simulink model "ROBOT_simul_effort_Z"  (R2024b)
settings: Solver=VariableStepAuto  StartTime=0.0  StopTime=5  RelTol=1e-3
undefined symbols (not defined in the file): a, ARRIERE_Defaut_sldprt, avant01_Defaut_sldprt, avant02_Defaut_sldprt, avant03_Defaut_sldprt, avant1_Defaut_sldprt, AXE, BASE_Defaut_sldprt, BIELLE, BIELLE_Defaut_sldprt, BRAS_Defaut_sldprt, bras_Defaut_sldprt, C_Realiste_sldprt, CABLE_Defaut_sldprt, cable_Defaut_sldprt, CACHE_Defaut_sldprt, CARTE, carte_Defaut_sldprt, CARTER, carter, CHC, CODEUR_Defaut_sldprt, cruciforme, cylindrique, deg, Drive, Fichiers, Fichiers_Matlab_sujetA, FIXATION, fixation_Defaut_sldprt, H, HEXAGONALE_Defaut_sldprt, joint_Defaut_sldprt, kg, m, M4, M4_Defaut_sldprt, manette1_Defaut_sldprt, manette2_Defaut_sldprt, MATLAB, Matlab, matlab_Defaut_sldprt, mm, modif, MOTEUR_Defaut_sldprt, N, NEZ_Defaut_sldprt, nom, palier, PARALLELOGRAMME_Defaut_sldprt, petite, plaque, rad, Ressort, Rondelle, ROTOR_Defaut_sldprt, s, SET, simple, socle_Defaut_sldprt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
libraries: sm_lib x463, fl_lib x45, nesl_utility x27, simulink x2
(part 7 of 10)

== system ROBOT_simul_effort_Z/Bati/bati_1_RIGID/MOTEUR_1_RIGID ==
  ReferenceFrame : sm_lib/Frames and Transforms/Reference Frame
  Solid : sm_lib/Body Elements/File Solid  ExtGeomFileName=/MATLAB Drive/Fichiers_Matlab_sujetA/Fichiers Matlab/STL/MOTEUR_Defaut_sldprt.STL  UnitType=Custom  ExtGeomFileUnits=mm  StepReaderType=HEX  ExportConvexHullGeometry=off  InertiaType=Custom  BasedOnType=Density  Density=1000  DensityUnits=kg/(m^3)  Mass=0.064287172119754279  MassUnits=kg  CenterOfMass=[0 32.927342518193171 0]  CenterOfMassUnits=mm  MomentsOfInertia=[23.361167142247837 11.499741081133124 23.353822804254591]  MomentsOfInertiaUnits=kg*mm^2  ProductsOfInertia=[0 0 0]  ProductsOfInertiaUnits=kg*mm^2  GraphicType=FromGeometry  MarkerShape=Sphere  MarkerSize=10  GraphicVisPropType=SimpleVisualProperties  GraphicDiffuseColor=[0.792156862745098 0.81960784313725488 0.93333333333333335]  GraphicOpacity=1  GraphicSpecularColor=[0.5 0.5 0.5 1.0]  GraphicAmbientColor=[0.15 0.15 0.15 1.0]  GraphicEmissiveColor=[0.0 0.0 0.0 1.0]  GraphicShininess=75  DoExposeReferenceFrame=on  SerializedFrames=<Frames/>
  F : PMIOPort  Side=Left
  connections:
  Solid/RConn1 -- ReferenceFrame/RConn1 -- F/RConn1

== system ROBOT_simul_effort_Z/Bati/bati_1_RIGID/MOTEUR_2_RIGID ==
  ReferenceFrame : sm_lib/Frames and Transforms/Reference Frame
  Solid : sm_lib/Body Elements/File Solid  ExtGeomFileName=/MATLAB Drive/Fichiers_Matlab_sujetA/Fichiers Matlab/STL/MOTEUR_Defaut_sldprt.STL  UnitType=Custom  ExtGeomFileUnits=mm  StepReaderType=HEX  ExportConvexHullGeometry=off  InertiaType=Custom  BasedOnType=Density  Density=1000  DensityUnits=kg/(m^3)  Mass=0.064287172119754279  MassUnits=kg  CenterOfMass=[0 32.927342518193171 0]  CenterOfMassUnits=mm  MomentsOfInertia=[23.361167142247837 11.499741081133124 23.353822804254591]  MomentsOfInertiaUnits=kg*mm^2  ProductsOfInertia=[0 0 0]  ProductsOfInertiaUnits=kg*mm^2  GraphicType=FromGeometry  MarkerShape=Sphere  MarkerSize=10  GraphicVisPropType=SimpleVisualProperties  GraphicDiffuseColor=[0.792156862745098 0.81960784313725488 0.93333333333333335]  GraphicOpacity=1  GraphicSpecularColor=[0.5 0.5 0.5 1.0]  GraphicAmbientColor=[0.15 0.15 0.15 1.0]  GraphicEmissiveColor=[0.0 0.0 0.0 1.0]  GraphicShininess=75  DoExposeReferenceFrame=on  SerializedFrames=<Frames/>
  F : PMIOPort  Side=Left
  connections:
  Solid/RConn1 -- ReferenceFrame/RConn1 -- F/RConn1

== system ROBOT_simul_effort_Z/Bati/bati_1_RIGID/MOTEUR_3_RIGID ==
  ReferenceFrame : sm_lib/Frames and Transforms/Reference Frame
  Solid : sm_lib/Body Elements/File Solid  ExtGeomFileName=/MATLAB Drive/Fichiers_Matlab_sujetA/Fichiers Matlab/STL/MOTEUR_Defaut_sldprt.STL  UnitType=Custom  ExtGeomFileUnits=mm  StepReaderType=HEX  ExportConvexHullGeometry=off  InertiaType=Custom  BasedOnType=Density  Density=1000  DensityUnits=kg/(m^3)  Mass=0.064287172119754279  MassUnits=kg  CenterOfMass=[0 32.927342518193171 0]  CenterOfMassUnits=mm  MomentsOfInertia=[23.361167142247837 11.499741081133124 23.353822804254591]  MomentsOfInertiaUnits=kg*mm^2  ProductsOfInertia=[0 0 0]  ProductsOfInertiaUnits=kg*mm^2  GraphicType=FromGeometry  MarkerShape=Sphere  MarkerSize=10  GraphicVisPropType=SimpleVisualProperties  GraphicDiffuseColor=[0.792156862745098 0.81960784313725488 0.93333333333333335]  GraphicOpacity=1  GraphicSpecularColor=[0.5 0.5 0.5 1.0]  GraphicAmbientColor=[0.15 0.15 0.15 1.0]  GraphicEmissiveColor=[0.0 0.0 0.0 1.0]  GraphicShininess=75  DoExposeReferenceFrame=on  SerializedFrames=<Frames/>
  F : PMIOPort  Side=Left
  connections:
  Solid/RConn1 -- ReferenceFrame/RConn1 -- F/RConn1

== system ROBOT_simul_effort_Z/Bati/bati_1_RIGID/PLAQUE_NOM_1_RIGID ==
  ReferenceFrame : sm_lib/Frames and Transforms/Reference Frame
  Solid : sm_lib/Body Elements/File Solid  ExtGeomFileName=/MATLAB Drive/Fichiers_Matlab_sujetA/Fichiers Matlab/STL/plaque nom simple-1.STL  UnitType=Custom  ExtGeomFileUnits=mm  StepReaderType=HEX  ExportConvexHullGeometry=off  InertiaType=Custom  BasedOnType=Density  Density=1000  DensityUnits=kg/(m^3)  Mass=0.00027200040900533893  MassUnits=kg  CenterOfMass=[-0.0026353545106053435 115.22134035146432 0.049293923597036424]  CenterOfMassUnits=mm  MomentsOfInertia=[0.063569474995042688 0.063782951879047547 0.12735197367307241]  MomentsOfInertiaUnits=kg*mm^2  ProductsOfInertia=[2.9045793709905346e-07 6.1711886469806189e-08 2.2164861893284939e-05]  ProductsOfInertiaUnits=kg*mm^2  GraphicType=FromGeometry  MarkerShape=Sphere  MarkerSize=10  GraphicVisPropType=SimpleVisualProperties  GraphicDiffuseColor=[1.0 1.0 1.0]  GraphicOpacity=1  GraphicSpecularColor=[0.5 0.5 0.5 1.0]  GraphicAmbientColor=[0.15 0.15 0.15 1.0]  GraphicEmissiveColor=[0.0 0.0 0.0 1.0]  GraphicShininess=75  DoExposeReferenceFrame=on  SerializedFrames=<Frames/>
  F : PMIOPort  Side=Left
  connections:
  Solid/RConn1 -- ReferenceFrame/RConn1 -- F/RConn1

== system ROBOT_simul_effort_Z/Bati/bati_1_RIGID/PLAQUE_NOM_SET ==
  ReferenceFrame : sm_lib/Frames and Transforms/Reference Frame
  Solid : sm_lib/Body Elements/File Solid  ExtGeomFileName=/MATLAB Drive/Fichiers_Matlab_sujetA/Fichiers Matlab/STL/plaque nom SET-1.STL  UnitType=Custom  ExtGeomFileUnits=mm  StepReaderType=HEX  ExportConvexHullGeometry=off  InertiaType=Custom  BasedOnType=Density  Density=1000  DensityUnits=kg/(m^3)  Mass=0.00027200040900533893  MassUnits=kg  CenterOfMass=[-0.0026353545106053435 115.22134035146432 0.049293923597036424]  CenterOfMassUnits=mm  MomentsOfInertia=[0.063569474995042688 0.063782951879047547 0.12735197367307241]  MomentsOfInertiaUnits=kg*mm^2  ProductsOfInertia=[2.9045793709905346e-07 6.1711886469806189e-08 2.2164861893284939e-05]  ProductsOfInertiaUnits=kg*mm^2  GraphicType=FromGeometry  MarkerShape=Sphere  MarkerSize=10  GraphicVisPropType=SimpleVisualProperties  GraphicDiffuseColor=[0.2 0.2 1.0]  GraphicOpacity=1  GraphicSpecularColor=[0.5 0.5 0.5 1.0]  GraphicAmbientColor=[0.15 0.15 0.15 1.0]  GraphicEmissiveColor=[0.0 0.0 0.0 1.0]  GraphicShininess=75  DoExposeReferenceFrame=on  SerializedFrames=<Frames/>
  F : PMIOPort  Side=Left
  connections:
  F/RConn1 -- ReferenceFrame/RConn1 -- Solid/RConn1

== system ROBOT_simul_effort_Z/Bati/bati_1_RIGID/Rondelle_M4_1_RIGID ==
  ReferenceFrame : sm_lib/Frames and Transforms/Reference Frame
  Solid : sm_lib/Body Elements/File Solid  ExtGeomFileName=/MATLAB Drive/Fichiers_Matlab_sujetA/Fichiers Matlab/STL/Rondelle M4_Defaut_sldprt.STL  UnitType=Custom  ExtGeomFileUnits=mm  StepReaderType=HEX  ExportConvexHullGeometry=off  InertiaType=Custom  BasedOnType=Density  Density=1000  DensityUnits=kg/(m^3)  Mass=4.0840704496667297e-05  MassUnits=kg  CenterOfMass=[0 0.39999999999999991 0]  CenterOfMassUnits=mm  MomentsOfInertia=[0.00024977494191753434 0.00049519354202209084 0.00024977494191753439]  MomentsOfInertiaUnits=kg*mm^2  ProductsOfInertia=[0 0 0]  ProductsOfInertiaUnits=kg*mm^2  GraphicType=FromGeometry  MarkerShape=Sphere  MarkerSize=10  GraphicVisPropType=SimpleVisualProperties  GraphicDiffuseColor=[0.792156862745098 0.81960784313725488 0.93333333333333335]  GraphicOpacity=1  GraphicSpecularColor=[0.5 0.5 0.5 1.0]  GraphicAmbientColor=[0.15 0.15 0.15 1.0]  GraphicEmissiveColor=[0.0 0.0 0.0 1.0]  GraphicShininess=75  DoExposeReferenceFrame=on  SerializedFrames=<Frames/>
  F : PMIOPort  Side=Left
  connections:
  Solid/RConn1 -- ReferenceFrame/RConn1 -- F/RConn1

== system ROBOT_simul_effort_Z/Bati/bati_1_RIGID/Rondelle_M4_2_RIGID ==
  ReferenceFrame : sm_lib/Frames and Transforms/Reference Frame
  Solid : sm_lib/Body Elements/File Solid  ExtGeomFileName=/MATLAB Drive/Fichiers_Matlab_sujetA/Fichiers Matlab/STL/Rondelle M4_Defaut_sldprt.STL  UnitType=Custom  ExtGeomFileUnits=mm  StepReaderType=HEX  ExportConvexHullGeometry=off  InertiaType=Custom  BasedOnType=Density  Density=1000  DensityUnits=kg/(m^3)  Mass=4.0840704496667297e-05  MassUnits=kg  CenterOfMass=[0 0.39999999999999991 0]  CenterOfMassUnits=mm  MomentsOfInertia=[0.00024977494191753434 0.00049519354202209084 0.00024977494191753439]  MomentsOfInertiaUnits=kg*mm^2  ProductsOfInertia=[0 0 0]  ProductsOfInertiaUnits=kg*mm^2  GraphicType=FromGeometry  MarkerShape=Sphere  MarkerSize=10  GraphicVisPropType=SimpleVisualProperties  GraphicDiffuseColor=[0.792156862745098 0.81960784313725488 0.93333333333333335]  GraphicOpacity=1  GraphicSpecularColor=[0.5 0.5 0.5 1.0]  GraphicAmbientColor=[0.15 0.15 0.15 1.0]  GraphicEmissiveColor=[0.0 0.0 0.0 1.0]  GraphicShininess=75  DoExposeReferenceFrame=on  SerializedFrames=<Frames/>
  F : PMIOPort  Side=Left
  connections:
  Solid/RConn1 -- ReferenceFrame/RConn1 -- F/RConn1

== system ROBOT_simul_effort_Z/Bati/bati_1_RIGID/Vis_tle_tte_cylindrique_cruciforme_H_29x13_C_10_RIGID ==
  ReferenceFrame : sm_lib/Frames and Transforms/Reference Frame
  Solid : sm_lib/Body Elements/File Solid  ExtGeomFileName=/MATLAB Drive/Fichiers_Matlab_sujetA/Fichiers Matlab/STL/Vis a tole tete cylindrique cruciforme H 2-9x13 - C_Realiste_sldprt.STL  UnitType=Custom  ExtGeomFileUnits=mm  StepReaderType=HEX  ExportConvexHullGeometry=off  InertiaType=Custom  BasedOnType=Density  Density=1000  DensityUnits=kg/(m^3)  Mass=8.3821869835456372e-05  MassUnits=kg  CenterOfMass=[4.9478681581074904 0.00064910481891303923 -0.0013634218224953438]  CenterOfMassUnits=mm  MomentsOfInertia=[0.00016543197172893975 0.0014334630955093895 0.0014333390308476422]  MomentsOfInertiaUnits=kg*mm^2  ProductsOfInertia=[-5.4062904633677868e-09 -1.3111174919527308e-07 6.0713893531177014e-07]  ProductsOfInertiaUnits=kg*mm^2  GraphicType=FromGeometry  MarkerShape=Sphere  MarkerSize=10  GraphicVisPropType=SimpleVisualProperties  GraphicDiffuseColor=[0.75294117647058822 0.75294117647058822 0.75294117647058822]  GraphicOpacity=1  GraphicSpecularColor=[0.5 0.5 0.5 1.0]  GraphicAmbientColor=[0.15 0.15 0.15 1.0]  GraphicEmissiveColor=[0.0 0.0 0.0 1.0]  GraphicShininess=75  DoExposeReferenceFrame=on  SerializedFrames=<Frames/>
  F : PMIOPort  Side=Left
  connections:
  Solid/RConn1 -- ReferenceFrame/RConn1 -- F/RConn1

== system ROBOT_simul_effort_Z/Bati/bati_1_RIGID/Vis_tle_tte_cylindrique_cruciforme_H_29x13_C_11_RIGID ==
  ReferenceFrame : sm_lib/Frames and Transforms/Reference Frame
  Solid : sm_lib/Body Elements/File Solid  ExtGeomFileName=/MATLAB Drive/Fichiers_Matlab_sujetA/Fichiers Matlab/STL/Vis a tole tete cylindrique cruciforme H 2-9x13 - C_Realiste_sldprt.STL  UnitType=Custom  ExtGeomFileUnits=mm  StepReaderType=HEX  ExportConvexHullGeometry=off  InertiaType=Custom  BasedOnType=Density  Density=1000  DensityUnits=kg/(m^3)  Mass=8.3821869835456372e-05  MassUnits=kg  CenterOfMass=[4.9478681581074904 0.00064910481891303923 -0.0013634218224953438]  CenterOfMassUnits=mm  MomentsOfInertia=[0.00016543197172893975 0.0014334630955093895 0.0014333390308476422]  MomentsOfInertiaUnits=kg*mm^2  ProductsOfInertia=[-5.4062904633677868e-09 -1.3111174919527308e-07 6.0713893531177014e-07]  ProductsOfInertiaUnits=kg*mm^2  GraphicType=FromGeometry  MarkerShape=Sphere  MarkerSize=10  GraphicVisPropType=SimpleVisualProperties  GraphicDiffuseColor=[0.75294117647058822 0.75294117647058822 0.75294117647058822]  GraphicOpacity=1  GraphicSpecularColor=[0.5 0.5 0.5 1.0]  GraphicAmbientColor=[0.15 0.15 0.15 1.0]  GraphicEmissiveColor=[0.0 0.0 0.0 1.0]  GraphicShininess=75  DoExposeReferenceFrame=on  SerializedFrames=<Frames/>
  F : PMIOPort  Side=Left
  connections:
  Solid/RConn1 -- ReferenceFrame/RConn1 -- F/RConn1

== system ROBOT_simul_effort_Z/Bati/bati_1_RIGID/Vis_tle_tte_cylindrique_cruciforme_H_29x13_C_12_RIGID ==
  ReferenceFrame : sm_lib/Frames and Transforms/Reference Frame
  Solid : sm_lib/Body Elements/File Solid  ExtGeomFileName=/MATLAB Drive/Fichiers_Matlab_sujetA/Fichiers Matlab/STL/Vis a tole tete cylindrique cruciforme H 2-9x13 - C_Realiste_sldprt.STL  UnitType=Custom  ExtGeomFileUnits=mm  StepReaderType=HEX  ExportConvexHullGeometry=off  InertiaType=Custom  BasedOnType=Density  Density=1000  DensityUnits=kg/(m^3)  Mass=8.3821869835456372e-05  MassUnits=kg  CenterOfMass=[4.9478681581074904 0.00064910481891303923 -0.0013634218224953438]  CenterOfMassUnits=mm  MomentsOfInertia=[0.00016543197172893975 0.0014334630955093895 0.0014333390308476422]  MomentsOfInertiaUnits=kg*mm^2  ProductsOfInertia=[-5.4062904633677868e-09 -1.3111174919527308e-07 6.0713893531177014e-07]  ProductsOfInertiaUnits=kg*mm^2  GraphicType=FromGeometry  MarkerShape=Sphere  MarkerSize=10  GraphicVisPropType=SimpleVisualProperties  GraphicDiffuseColor=[0.75294117647058822 0.75294117647058822 0.75294117647058822]  GraphicOpacity=1  GraphicSpecularColor=[0.5 0.5 0.5 1.0]  GraphicAmbientColor=[0.15 0.15 0.15 1.0]  GraphicEmissiveColor=[0.0 0.0 0.0 1.0]  GraphicShininess=75  DoExposeReferenceFrame=on  SerializedFrames=<Frames/>
  F : PMIOPort  Side=Left
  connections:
  Solid/RConn1 -- ReferenceFrame/RConn1 -- F/RConn1

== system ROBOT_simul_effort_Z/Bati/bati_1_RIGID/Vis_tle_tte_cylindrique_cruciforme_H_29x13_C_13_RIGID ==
  ReferenceFrame : sm_lib/Frames and Transforms/Reference Frame
  Solid : sm_lib/Body Elements/File Solid  ExtGeomFileName=/MATLAB Drive/Fichiers_Matlab_sujetA/Fichiers Matlab/STL/Vis a tole tete cylindrique cruciforme H 2-9x13 - C_Realiste_sldprt.STL  UnitType=Custom  ExtGeomFileUnits=mm  StepReaderType=HEX  ExportConvexHullGeometry=off  InertiaType=Custom  BasedOnType=Density  Density=1000  DensityUnits=kg/(m^3)  Mass=8.3821869835456372e-05  MassUnits=kg  CenterOfMass=[4.9478681581074904 0.00064910481891303923 -0.0013634218224953438]  CenterOfMassUnits=mm  MomentsOfInertia=[0.00016543197172893975 0.0014334630955093895 0.0014333390308476422]  MomentsOfInertiaUnits=kg*mm^2  ProductsOfInertia=[-5.4062904633677868e-09 -1.3111174919527308e-07 6.0713893531177014e-07]  ProductsOfInertiaUnits=kg*mm^2  GraphicType=FromGeometry  MarkerShape=Sphere  MarkerSize=10  GraphicVisPropType=SimpleVisualProperties  GraphicDiffuseColor=[0.75294117647058822 0.75294117647058822 0.75294117647058822]  GraphicOpacity=1  GraphicSpecularColor=[0.5 0.5 0.5 1.0]  GraphicAmbientColor=[0.15 0.15 0.15 1.0]  GraphicEmissiveColor=[0.0 0.0 0.0 1.0]  GraphicShininess=75  DoExposeReferenceFrame=on  SerializedFrames=<Frames/>
  F : PMIOPort  Side=Left
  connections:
  Solid/RConn1 -- ReferenceFrame/RConn1 -- F/RConn1

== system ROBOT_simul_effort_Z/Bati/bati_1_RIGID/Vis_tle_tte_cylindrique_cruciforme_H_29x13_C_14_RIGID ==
  ReferenceFrame : sm_lib/Frames and Transforms/Reference Frame
  Solid : sm_lib/Body Elements/File Solid  ExtGeomFileName=/MATLAB Drive/Fichiers_Matlab_sujetA/Fichiers Matlab/STL/Vis a tole tete cylindrique cruciforme H 2-9x13 - C_Realiste_sldprt.STL  UnitType=Custom  ExtGeomFileUnits=mm  StepReaderType=HEX  ExportConvexHullGeometry=off  InertiaType=Custom  BasedOnType=Density  Density=1000  DensityUnits=kg/(m^3)  Mass=8.3821869835456372e-05  MassUnits=kg  CenterOfMass=[4.9478681581074904 0.00064910481891303923 -0.0013634218224953438]  CenterOfMassUnits=mm  MomentsOfInertia=[0.00016543197172893975 0.0014334630955093895 0.0014333390308476422]  MomentsOfInertiaUnits=kg*mm^2  ProductsOfInertia=[-5.4062904633677868e-09 -1.3111174919527308e-07 6.0713893531177014e-07]  ProductsOfInertiaUnits=kg*mm^2  GraphicType=FromGeometry  MarkerShape=Sphere  MarkerSize=10  GraphicVisPropType=SimpleVisualProperties  GraphicDiffuseColor=[0.75294117647058822 0.75294117647058822 0.75294117647058822]  GraphicOpacity=1  GraphicSpecularColor=[0.5 0.5 0.5 1.0]  GraphicAmbientColor=[0.15 0.15 0.15 1.0]  GraphicEmissiveColor=[0.0 0.0 0.0 1.0]  GraphicShininess=75  DoExposeReferenceFrame=on  SerializedFrames=<Frames/>
  F : PMIOPort  Side=Left
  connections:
  Solid/RConn1 -- ReferenceFrame/RConn1 -- F/RConn1

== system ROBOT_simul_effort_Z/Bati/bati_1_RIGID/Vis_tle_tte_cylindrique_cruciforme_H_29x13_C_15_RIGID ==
  ReferenceFrame : sm_lib/Frames and Transforms/Reference Frame
  Solid : sm_lib/Body Elements/File Solid  ExtGeomFileName=/MATLAB Drive/Fichiers_Matlab_sujetA/Fichiers Matlab/STL/Vis a tole tete cylindrique cruciforme H 2-9x13 - C_Realiste_sldprt.STL  UnitType=Custom  ExtGeomFileUnits=mm  StepReaderType=HEX  ExportConvexHullGeometry=off  InertiaType=Custom  BasedOnType=Density  Density=1000  DensityUnits=kg/(m^3)  Mass=8.3821869835456372e-05  MassUnits=kg  CenterOfMass=[4.9478681581074904 0.00064910481891303923 -0.0013634218224953438]  CenterOfMassUnits=mm  MomentsOfInertia=[0.00016543197172893975 0.0014334630955093895 0.0014333390308476422]  MomentsOfInertiaUnits=kg*mm^2  ProductsOfInertia=[-5.4062904633677868e-09 -1.3111174919527308e-07 6.0713893531177014e-07]  ProductsOfInertiaUnits=kg*mm^2  GraphicType=FromGeometry  MarkerShape=Sphere  MarkerSize=10  GraphicVisPropType=SimpleVisualProperties  GraphicDiffuseColor=[0.75294117647058822 0.75294117647058822 0.75294117647058822]  GraphicOpacity=1  GraphicSpecularColor=[0.5 0.5 0.5 1.0]  GraphicAmbientColor=[0.15 0.15 0.15 1.0]  GraphicEmissiveColor=[0.0 0.0 0.0 1.0]  GraphicShininess=75  DoExposeReferenceFrame=on  SerializedFrames=<Frames/>
  F : PMIOPort  Side=Left
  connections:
  Solid/RConn1 -- ReferenceFrame/RConn1 -- F/RConn1

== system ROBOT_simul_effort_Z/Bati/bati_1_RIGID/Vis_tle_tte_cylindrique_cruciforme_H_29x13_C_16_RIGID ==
  ReferenceFrame : sm_lib/Frames and Transforms/Reference Frame
  Solid : sm_lib/Body Elements/File Solid  ExtGeomFileName=/MATLAB Drive/Fichiers_Matlab_sujetA/Fichiers Matlab/STL/Vis a tole tete cylindrique cruciforme H 2-9x13 - C_Realiste_sldprt.STL  UnitType=Custom  ExtGeomFileUnits=mm  StepReaderType=HEX  ExportConvexHullGeometry=off  InertiaType=Custom  BasedOnType=Density  Density=1000  DensityUnits=kg/(m^3)  Mass=8.3821869835456372e-05  MassUnits=kg  CenterOfMass=[4.9478681581074904 0.00064910481891303923 -0.0013634218224953438]  CenterOfMassUnits=mm  MomentsOfInertia=[0.00016543197172893975 0.0014334630955093895 0.0014333390308476422]  MomentsOfInertiaUnits=kg*mm^2  ProductsOfInertia=[-5.4062904633677868e-09 -1.3111174919527308e-07 6.0713893531177014e-07]  ProductsOfInertiaUnits=kg*mm^2  GraphicType=FromGeometry  MarkerShape=Sphere  MarkerSize=10  GraphicVisPropType=SimpleVisualProperties  GraphicDiffuseColor=[0.75294117647058822 0.75294117647058822 0.75294117647058822]  GraphicOpacity=1  GraphicSpecularColor=[0.5 0.5 0.5 1.0]  GraphicAmbientColor=[0.15 0.15 0.15 1.0]  GraphicEmissiveColor=[0.0 0.0 0.0 1.0]  GraphicShininess=75  DoExposeReferenceFrame=on  SerializedFrames=<Frames/>
  F : PMIOPort  Side=Left
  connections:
  Solid/RConn1 -- ReferenceFrame/RConn1 -- F/RConn1

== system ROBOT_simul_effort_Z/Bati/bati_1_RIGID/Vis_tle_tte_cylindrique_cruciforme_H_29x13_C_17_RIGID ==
  ReferenceFrame : sm_lib/Frames and Transforms/Reference Frame
  Solid : sm_lib/Body Elements/File Solid  ExtGeomFileName=/MATLAB Drive/Fichiers_Matlab_sujetA/Fichiers Matlab/STL/Vis a tole tete cylindrique cruciforme H 2-9x13 - C_Realiste_sldprt.STL  UnitType=Custom  ExtGeomFileUnits=mm  StepReaderType=HEX  ExportConvexHullGeometry=off  InertiaType=Custom  BasedOnType=Density  Density=1000  DensityUnits=kg/(m^3)  Mass=8.3821869835456372e-05  MassUnits=kg  CenterOfMass=[4.9478681581074904 0.00064910481891303923 -0.0013634218224953438]  CenterOfMassUnits=mm  MomentsOfInertia=[0.00016543197172893975 0.0014334630955093895 0.0014333390308476422]  MomentsOfInertiaUnits=kg*mm^2  ProductsOfInertia=[-5.4062904633677868e-09 -1.3111174919527308e-07 6.0713893531177014e-07]  ProductsOfInertiaUnits=kg*mm^2  GraphicType=FromGeometry  MarkerShape=Sphere  MarkerSize=10  GraphicVisPropType=SimpleVisualProperties  GraphicDiffuseColor=[0.75294117647058822 0.75294117647058822 0.75294117647058822]  GraphicOpacity=1  GraphicSpecularColor=[0.5 0.5 0.5 1.0]  GraphicAmbientColor=[0.15 0.15 0.15 1.0]  GraphicEmissiveColor=[0.0 0.0 0.0 1.0]  GraphicShininess=75  DoExposeReferenceFrame=on  SerializedFrames=<Frames/>
  F : PMIOPort  Side=Left
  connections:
  Solid/RConn1 -- ReferenceFrame/RConn1 -- F/RConn1

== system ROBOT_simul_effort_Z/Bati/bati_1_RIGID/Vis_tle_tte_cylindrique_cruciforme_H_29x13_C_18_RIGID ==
  ReferenceFrame : sm_lib/Frames and Transforms/Reference Frame
  Solid : sm_lib/Body Elements/File Solid  ExtGeomFileName=/MATLAB Drive/Fichiers_Matlab_sujetA/Fichiers Matlab/STL/Vis a tole tete cylindrique cruciforme H 2-9x13 - C_Realiste_sldprt.STL  UnitType=Custom  ExtGeomFileUnits=mm  StepReaderType=HEX  ExportConvexHullGeometry=off  InertiaType=Custom  BasedOnType=Density  Density=1000  DensityUnits=kg/(m^3)  Mass=8.3821869835456372e-05  MassUnits=kg  CenterOfMass=[4.9478681581074904 0.00064910481891303923 -0.0013634218224953438]  CenterOfMassUnits=mm  MomentsOfInertia=[0.00016543197172893975 0.0014334630955093895 0.0014333390308476422]  MomentsOfInertiaUnits=kg*mm^2  ProductsOfInertia=[-5.4062904633677868e-09 -1.3111174919527308e-07 6.0713893531177014e-07]  ProductsOfInertiaUnits=kg*mm^2  GraphicType=FromGeometry  MarkerShape=Sphere  MarkerSize=10  GraphicVisPropType=SimpleVisualProperties  GraphicDiffuseColor=[0.75294117647058822 0.75294117647058822 0.75294117647058822]  GraphicOpacity=1  GraphicSpecularColor=[0.5 0.5 0.5 1.0]  GraphicAmbientColor=[0.15 0.15 0.15 1.0]  GraphicEmissiveColor=[0.0 0.0 0.0 1.0]  GraphicShininess=75  DoExposeReferenceFrame=on  SerializedFrames=<Frames/>
  F : PMIOPort  Side=Left
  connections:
  Solid/RConn1 -- ReferenceFrame/RConn1 -- F/RConn1

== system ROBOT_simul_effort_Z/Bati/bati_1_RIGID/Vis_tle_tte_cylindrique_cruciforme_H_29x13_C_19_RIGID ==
  ReferenceFrame : sm_lib/Frames and Transforms/Reference Frame
  Solid : sm_lib/Body Elements/File Solid  ExtGeomFileName=/MATLAB Drive/Fichiers_Matlab_sujetA/Fichiers Matlab/STL/Vis a tole tete cylindrique cruciforme H 2-9x13 - C_Realiste_sldprt.STL  UnitType=Custom  ExtGeomFileUnits=mm  StepReaderType=HEX  ExportConvexHullGeometry=off  InertiaType=Custom  BasedOnType=Density  Density=1000  DensityUnits=kg/(m^3)  Mass=8.3821869835456372e-05  MassUnits=kg  CenterOfMass=[4.9478681581074904 0.00064910481891303923 -0.0013634218224953438]  CenterOfMassUnits=mm  MomentsOfInertia=[0.00016543197172893975 0.0014334630955093895 0.0014333390308476422]  MomentsOfInertiaUnits=kg*mm^2  ProductsOfInertia=[-5.4062904633677868e-09 -1.3111174919527308e-07 6.0713893531177014e-07]  ProductsOfInertiaUnits=kg*mm^2  GraphicType=FromGeometry  MarkerShape=Sphere  MarkerSize=10  GraphicVisPropType=SimpleVisualProperties  GraphicDiffuseColor=[0.75294117647058822 0.75294117647058822 0.75294117647058822]  GraphicOpacity=1  GraphicSpecularColor=[0.5 0.5 0.5 1.0]  GraphicAmbientColor=[0.15 0.15 0.15 1.0]  GraphicEmissiveColor=[0.0 0.0 0.0 1.0]  GraphicShininess=75  DoExposeReferenceFrame=on  SerializedFrames=<Frames/>
  F : PMIOPort  Side=Left
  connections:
  Solid/RConn1 -- ReferenceFrame/RConn1 -- F/RConn1

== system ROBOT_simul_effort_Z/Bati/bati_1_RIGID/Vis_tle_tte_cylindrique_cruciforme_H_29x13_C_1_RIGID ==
  ReferenceFrame : sm_lib/Frames and Transforms/Reference Frame
  Solid : sm_lib/Body Elements/File Solid  ExtGeomFileName=/MATLAB Drive/Fichiers_Matlab_sujetA/Fichiers Matlab/STL/Vis a tole tete cylindrique cruciforme H 2-9x13 - C_Realiste_sldprt.STL  UnitType=Custom  ExtGeomFileUnits=mm  StepReaderType=HEX  ExportConvexHullGeometry=off  InertiaType=Custom  BasedOnType=Density  Density=1000  DensityUnits=kg/(m^3)  Mass=8.3821869835456372e-05  MassUnits=kg  CenterOfMass=[4.9478681581074904 0.00064910481891303923 -0.0013634218224953438]  CenterOfMassUnits=mm  MomentsOfInertia=[0.00016543197172893975 0.0014334630955093895 0.0014333390308476422]  MomentsOfInertiaUnits=kg*mm^2  ProductsOfInertia=[-5.4062904633677868e-09 -1.3111174919527308e-07 6.0713893531177014e-07]  ProductsOfInertiaUnits=kg*mm^2  GraphicType=FromGeometry  MarkerShape=Sphere  MarkerSize=10  GraphicVisPropType=SimpleVisualProperties  GraphicDiffuseColor=[0.75294117647058822 0.75294117647058822 0.75294117647058822]  GraphicOpacity=1  GraphicSpecularColor=[0.5 0.5 0.5 1.0]  GraphicAmbientColor=[0.15 0.15 0.15 1.0]  GraphicEmissiveColor=[0.0 0.0 0.0 1.0]  GraphicShininess=75  DoExposeReferenceFrame=on  SerializedFrames=<Frames/>
  F : PMIOPort  Side=Left
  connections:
  Solid/RConn1 -- ReferenceFrame/RConn1 -- F/RConn1

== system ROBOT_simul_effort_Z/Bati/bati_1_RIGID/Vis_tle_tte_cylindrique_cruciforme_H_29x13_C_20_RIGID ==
  ReferenceFrame : sm_lib/Frames and Transforms/Reference Frame
  Solid : sm_lib/Body Elements/File Solid  ExtGeomFileName=/MATLAB Drive/Fichiers_Matlab_sujetA/Fichiers Matlab/STL/Vis a tole tete cylindrique cruciforme H 2-9x13 - C_Realiste_sldprt.STL  UnitType=Custom  ExtGeomFileUnits=mm  StepReaderType=HEX  ExportConvexHullGeometry=off  InertiaType=Custom  BasedOnType=Density  Density=1000  DensityUnits=kg/(m^3)  Mass=8.3821869835456372e-05  MassUnits=kg  CenterOfMass=[4.9478681581074904 0.00064910481891303923 -0.0013634218224953438]  CenterOfMassUnits=mm  MomentsOfInertia=[0.00016543197172893975 0.0014334630955093895 0.0014333390308476422]  MomentsOfInertiaUnits=kg*mm^2  ProductsOfInertia=[-5.4062904633677868e-09 -1.3111174919527308e-07 6.0713893531177014e-07]  ProductsOfInertiaUnits=kg*mm^2  GraphicType=FromGeometry  MarkerShape=Sphere  MarkerSize=10  GraphicVisPropType=SimpleVisualProperties  GraphicDiffuseColor=[0.75294117647058822 0.75294117647058822 0.75294117647058822]  GraphicOpacity=1  GraphicSpecularColor=[0.5 0.5 0.5 1.0]  GraphicAmbientColor=[0.15 0.15 0.15 1.0]  GraphicEmissiveColor=[0.0 0.0 0.0 1.0]  GraphicShininess=75  DoExposeReferenceFrame=on  SerializedFrames=<Frames/>
  F : PMIOPort  Side=Left
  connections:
  Solid/RConn1 -- ReferenceFrame/RConn1 -- F/RConn1

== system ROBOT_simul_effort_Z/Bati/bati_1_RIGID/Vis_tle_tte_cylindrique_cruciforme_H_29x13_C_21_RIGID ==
  ReferenceFrame : sm_lib/Frames and Transforms/Reference Frame
  Solid : sm_lib/Body Elements/File Solid  ExtGeomFileName=/MATLAB Drive/Fichiers_Matlab_sujetA/Fichiers Matlab/STL/Vis a tole tete cylindrique cruciforme H 2-9x13 - C_Realiste_sldprt.STL  UnitType=Custom  ExtGeomFileUnits=mm  StepReaderType=HEX  ExportConvexHullGeometry=off  InertiaType=Custom  BasedOnType=Density  Density=1000  DensityUnits=kg/(m^3)  Mass=8.3821869835456372e-05  MassUnits=kg  CenterOfMass=[4.9478681581074904 0.00064910481891303923 -0.0013634218224953438]  CenterOfMassUnits=mm  MomentsOfInertia=[0.00016543197172893975 0.0014334630955093895 0.0014333390308476422]  MomentsOfInertiaUnits=kg*mm^2  ProductsOfInertia=[-5.4062904633677868e-09 -1.3111174919527308e-07 6.0713893531177014e-07]  ProductsOfInertiaUnits=kg*mm^2  GraphicType=FromGeometry  MarkerShape=Sphere  MarkerSize=10  GraphicVisPropType=SimpleVisualProperties  GraphicDiffuseColor=[0.75294117647058822 0.75294117647058822 0.75294117647058822]  GraphicOpacity=1  GraphicSpecularColor=[0.5 0.5 0.5 1.0]  GraphicAmbientColor=[0.15 0.15 0.15 1.0]  GraphicEmissiveColor=[0.0 0.0 0.0 1.0]  GraphicShininess=75  DoExposeReferenceFrame=on  SerializedFrames=<Frames/>
  F : PMIOPort  Side=Left
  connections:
  Solid/RConn1 -- ReferenceFrame/RConn1 -- F/RConn1

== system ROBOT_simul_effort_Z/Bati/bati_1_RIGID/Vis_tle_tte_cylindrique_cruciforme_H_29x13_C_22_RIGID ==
  ReferenceFrame : sm_lib/Frames and Transforms/Reference Frame
  Solid : sm_lib/Body Elements/File Solid  ExtGeomFileName=/MATLAB Drive/Fichiers_Matlab_sujetA/Fichiers Matlab/STL/Vis a tole tete cylindrique cruciforme H 2-9x13 - C_Realiste_sldprt.STL  UnitType=Custom  ExtGeomFileUnits=mm  StepReaderType=HEX  ExportConvexHullGeometry=off  InertiaType=Custom  BasedOnType=Density  Density=1000  DensityUnits=kg/(m^3)  Mass=8.3821869835456372e-05  MassUnits=kg  CenterOfMass=[4.9478681581074904 0.00064910481891303923 -0.0013634218224953438]  CenterOfMassUnits=mm  MomentsOfInertia=[0.00016543197172893975 0.0014334630955093895 0.0014333390308476422]  MomentsOfInertiaUnits=kg*mm^2  ProductsOfInertia=[-5.4062904633677868e-09 -1.3111174919527308e-07 6.0713893531177014e-07]  ProductsOfInertiaUnits=kg*mm^2  GraphicType=FromGeometry  MarkerShape=Sphere  MarkerSize=10  GraphicVisPropType=SimpleVisualProperties  GraphicDiffuseColor=[0.75294117647058822 0.75294117647058822 0.75294117647058822]  GraphicOpacity=1  GraphicSpecularColor=[0.5 0.5 0.5 1.0]  GraphicAmbientColor=[0.15 0.15 0.15 1.0]  GraphicEmissiveColor=[0.0 0.0 0.0 1.0]  GraphicShininess=75  DoExposeReferenceFrame=on  SerializedFrames=<Frames/>
  F : PMIOPort  Side=Left
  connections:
  Solid/RConn1 -- ReferenceFrame/RConn1 -- F/RConn1

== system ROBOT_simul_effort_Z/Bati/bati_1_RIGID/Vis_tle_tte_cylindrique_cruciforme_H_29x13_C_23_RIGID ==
  ReferenceFrame : sm_lib/Frames and Transforms/Reference Frame
  Solid : sm_lib/Body Elements/File Solid  ExtGeomFileName=/MATLAB Drive/Fichiers_Matlab_sujetA/Fichiers Matlab/STL/Vis a tole tete cylindrique cruciforme H 2-9x13 - C_Realiste_sldprt.STL  UnitType=Custom  ExtGeomFileUnits=mm  StepReaderType=HEX  ExportConvexHullGeometry=off  InertiaType=Custom  BasedOnType=Density  Density=1000  DensityUnits=kg/(m^3)  Mass=8.3821869835456372e-05  MassUnits=kg  CenterOfMass=[4.9478681581074904 0.00064910481891303923 -0.0013634218224953438]  CenterOfMassUnits=mm  MomentsOfInertia=[0.00016543197172893975 0.0014334630955093895 0.0014333390308476422]  MomentsOfInertiaUnits=kg*mm^2  ProductsOfInertia=[-5.4062904633677868e-09 -1.3111174919527308e-07 6.0713893531177014e-07]  ProductsOfInertiaUnits=kg*mm^2  GraphicType=FromGeometry  MarkerShape=Sphere  MarkerSize=10  GraphicVisPropType=SimpleVisualProperties  GraphicDiffuseColor=[0.75294117647058822 0.75294117647058822 0.75294117647058822]  GraphicOpacity=1  GraphicSpecularColor=[0.5 0.5 0.5 1.0]  GraphicAmbientColor=[0.15 0.15 0.15 1.0]  GraphicEmissiveColor=[0.0 0.0 0.0 1.0]  GraphicShininess=75  DoExposeReferenceFrame=on  SerializedFrames=<Frames/>
  F : PMIOPort  Side=Left
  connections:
  Solid/RConn1 -- ReferenceFrame/RConn1 -- F/RConn1

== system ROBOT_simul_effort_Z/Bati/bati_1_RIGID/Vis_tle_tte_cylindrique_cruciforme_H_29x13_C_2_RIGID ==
  ReferenceFrame : sm_lib/Frames and Transforms/Reference Frame
  Solid : sm_lib/Body Elements/File Solid  ExtGeomFileName=/MATLAB Drive/Fichiers_Matlab_sujetA/Fichiers Matlab/STL/Vis a tole tete cylindrique cruciforme H 2-9x13 - C_Realiste_sldprt.STL  UnitType=Custom  ExtGeomFileUnits=mm  StepReaderType=HEX  ExportConvexHullGeometry=off  InertiaType=Custom  BasedOnType=Density  Density=1000  DensityUnits=kg/(m^3)  Mass=8.3821869835456372e-05  MassUnits=kg  CenterOfMass=[4.9478681581074904 0.00064910481891303923 -0.0013634218224953438]  CenterOfMassUnits=mm  MomentsOfInertia=[0.00016543197172893975 0.0014334630955093895 0.0014333390308476422]  MomentsOfInertiaUnits=kg*mm^2  ProductsOfInertia=[-5.4062904633677868e-09 -1.3111174919527308e-07 6.0713893531177014e-07]  ProductsOfInertiaUnits=kg*mm^2  GraphicType=FromGeometry  MarkerShape=Sphere  MarkerSize=10  GraphicVisPropType=SimpleVisualProperties  GraphicDiffuseColor=[0.75294117647058822 0.75294117647058822 0.75294117647058822]  GraphicOpacity=1  GraphicSpecularColor=[0.5 0.5 0.5 1.0]  GraphicAmbientColor=[0.15 0.15 0.15 1.0]  GraphicEmissiveColor=[0.0 0.0 0.0 1.0]  GraphicShininess=75  DoExposeReferenceFrame=on  SerializedFrames=<Frames/>
  F : PMIOPort  Side=Left
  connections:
  Solid/RConn1 -- ReferenceFrame/RConn1 -- F/RConn1

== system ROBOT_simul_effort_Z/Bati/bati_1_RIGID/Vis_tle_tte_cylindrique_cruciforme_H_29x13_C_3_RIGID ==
  ReferenceFrame : sm_lib/Frames and Transforms/Reference Frame
  Solid : sm_lib/Body Elements/File Solid  ExtGeomFileName=/MATLAB Drive/Fichiers_Matlab_sujetA/Fichiers Matlab/STL/Vis a tole tete cylindrique cruciforme H 2-9x13 - C_Realiste_sldprt.STL  UnitType=Custom  ExtGeomFileUnits=mm  StepReaderType=HEX  ExportConvexHullGeometry=off  InertiaType=Custom  BasedOnType=Density  Density=1000  DensityUnits=kg/(m^3)  Mass=8.3821869835456372e-05  MassUnits=kg  CenterOfMass=[4.9478681581074904 0.00064910481891303923 -0.0013634218224953438]  CenterOfMassUnits=mm  MomentsOfInertia=[0.00016543197172893975 0.0014334630955093895 0.0014333390308476422]  MomentsOfInertiaUnits=kg*mm^2  ProductsOfInertia=[-5.4062904633677868e-09 -1.3111174919527308e-07 6.0713893531177014e-07]  ProductsOfInertiaUnits=kg*mm^2  GraphicType=FromGeometry  MarkerShape=Sphere  MarkerSize=10  GraphicVisPropType=SimpleVisualProperties  GraphicDiffuseColor=[0.75294117647058822 0.75294117647058822 0.75294117647058822]  GraphicOpacity=1  GraphicSpecularColor=[0.5 0.5 0.5 1.0]  GraphicAmbientColor=[0.15 0.15 0.15 1.0]  GraphicEmissiveColor=[0.0 0.0 0.0 1.0]  GraphicShininess=75  DoExposeReferenceFrame=on  SerializedFrames=<Frames/>
  F : PMIOPort  Side=Left
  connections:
  Solid/RConn1 -- ReferenceFrame/RConn1 -- F/RConn1

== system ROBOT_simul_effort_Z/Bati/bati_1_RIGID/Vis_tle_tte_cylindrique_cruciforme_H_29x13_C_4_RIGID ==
  ReferenceFrame : sm_lib/Frames and Transforms/Reference Frame
  Solid : sm_lib/Body Elements/File Solid  ExtGeomFileName=/MATLAB Drive/Fichiers_Matlab_sujetA/Fichiers Matlab/STL/Vis a tole tete cylindrique cruciforme H 2-9x13 - C_Realiste_sldprt.STL  UnitType=Custom  ExtGeomFileUnits=mm  StepReaderType=HEX  ExportConvexHullGeometry=off  InertiaType=Custom  BasedOnType=Density  Density=1000  DensityUnits=kg/(m^3)  Mass=8.3821869835456372e-05  MassUnits=kg  CenterOfMass=[4.9478681581074904 0.00064910481891303923 -0.0013634218224953438]  CenterOfMassUnits=mm  MomentsOfInertia=[0.00016543197172893975 0.0014334630955093895 0.0014333390308476422]  MomentsOfInertiaUnits=kg*mm^2  ProductsOfInertia=[-5.4062904633677868e-09 -1.3111174919527308e-07 6.0713893531177014e-07]  ProductsOfInertiaUnits=kg*mm^2  GraphicType=FromGeometry  MarkerShape=Sphere  MarkerSize=10  GraphicVisPropType=SimpleVisualProperties  GraphicDiffuseColor=[0.75294117647058822 0.75294117647058822 0.75294117647058822]  GraphicOpacity=1  GraphicSpecularColor=[0.5 0.5 0.5 1.0]  GraphicAmbientColor=[0.15 0.15 0.15 1.0]  GraphicEmissiveColor=[0.0 0.0 0.0 1.0]  GraphicShininess=75  DoExposeReferenceFrame=on  SerializedFrames=<Frames/>
  F : PMIOPort  Side=Left
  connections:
  Solid/RConn1 -- ReferenceFrame/RConn1 -- F/RConn1

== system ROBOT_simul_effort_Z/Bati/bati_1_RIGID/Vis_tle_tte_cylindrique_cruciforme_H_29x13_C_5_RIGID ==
  ReferenceFrame : sm_lib/Frames and Transforms/Reference Frame
  Solid : sm_lib/Body Elements/File Solid  ExtGeomFileName=/MATLAB Drive/Fichiers_Matlab_sujetA/Fichiers Matlab/STL/Vis a tole tete cylindrique cruciforme H 2-9x13 - C_Realiste_sldprt.STL  UnitType=Custom  ExtGeomFileUnits=mm  StepReaderType=HEX  ExportConvexHullGeometry=off  InertiaType=Custom  BasedOnType=Density  Density=1000  DensityUnits=kg/(m^3)  Mass=8.3821869835456372e-05  MassUnits=kg  CenterOfMass=[4.9478681581074904 0.00064910481891303923 -0.0013634218224953438]  CenterOfMassUnits=mm  MomentsOfInertia=[0.00016543197172893975 0.0014334630955093895 0.0014333390308476422]  MomentsOfInertiaUnits=kg*mm^2  ProductsOfInertia=[-5.4062904633677868e-09 -1.3111174919527308e-07 6.0713893531177014e-07]  ProductsOfInertiaUnits=kg*mm^2  GraphicType=FromGeometry  MarkerShape=Sphere  MarkerSize=10  GraphicVisPropType=SimpleVisualProperties  GraphicDiffuseColor=[0.75294117647058822 0.75294117647058822 0.75294117647058822]  GraphicOpacity=1  GraphicSpecularColor=[0.5 0.5 0.5 1.0]  GraphicAmbientColor=[0.15 0.15 0.15 1.0]  GraphicEmissiveColor=[0.0 0.0 0.0 1.0]  GraphicShininess=75  DoExposeReferenceFrame=on  SerializedFrames=<Frames/>
  F : PMIOPort  Side=Left
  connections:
  Solid/RConn1 -- ReferenceFrame/RConn1 -- F/RConn1

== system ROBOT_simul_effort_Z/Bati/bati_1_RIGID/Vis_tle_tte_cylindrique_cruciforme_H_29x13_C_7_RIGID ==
  ReferenceFrame : sm_lib/Frames and Transforms/Reference Frame
  Solid : sm_lib/Body Elements/File Solid  ExtGeomFileName=/MATLAB Drive/Fichiers_Matlab_sujetA/Fichiers Matlab/STL/Vis a tole tete cylindrique cruciforme H 2-9x13 - C_Realiste_sldprt.STL  UnitType=Custom  ExtGeomFileUnits=mm  StepReaderType=HEX  ExportConvexHullGeometry=off  InertiaType=Custom  BasedOnType=Density  Density=1000  DensityUnits=kg/(m^3)  Mass=8.3821869835456372e-05  MassUnits=kg  CenterOfMass=[4.9478681581074904 0.00064910481891303923 -0.0013634218224953438]  CenterOfMassUnits=mm  MomentsOfInertia=[0.00016543197172893975 0.0014334630955093895 0.0014333390308476422]  MomentsOfInertiaUnits=kg*mm^2  ProductsOfInertia=[-5.4062904633677868e-09 -1.3111174919527308e-07 6.0713893531177014e-07]  ProductsOfInertiaUnits=kg*mm^2  GraphicType=FromGeometry  MarkerShape=Sphere  MarkerSize=10  GraphicVisPropType=SimpleVisualProperties  GraphicDiffuseColor=[0.75294117647058822 0.75294117647058822 0.75294117647058822]  GraphicOpacity=1  GraphicSpecularColor=[0.5 0.5 0.5 1.0]  GraphicAmbientColor=[0.15 0.15 0.15 1.0]  GraphicEmissiveColor=[0.0 0.0 0.0 1.0]  GraphicShininess=75  DoExposeReferenceFrame=on  SerializedFrames=<Frames/>
  F : PMIOPort  Side=Left
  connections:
  Solid/RConn1 -- ReferenceFrame/RConn1 -- F/RConn1

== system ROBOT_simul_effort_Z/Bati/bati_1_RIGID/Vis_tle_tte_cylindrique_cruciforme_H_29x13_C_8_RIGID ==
  ReferenceFrame : sm_lib/Frames and Transforms/Reference Frame
  Solid : sm_lib/Body Elements/File Solid  ExtGeomFileName=/MATLAB Drive/Fichiers_Matlab_sujetA/Fichiers Matlab/STL/Vis a tole tete cylindrique cruciforme H 2-9x13 - C_Realiste_sldprt.STL  UnitType=Custom  ExtGeomFileUnits=mm  StepReaderType=HEX  ExportConvexHullGeometry=off  InertiaType=Custom  BasedOnType=Density  Density=1000  DensityUnits=kg/(m^3)  Mass=8.3821869835456372e-05  MassUnits=kg  CenterOfMass=[4.9478681581074904 0.00064910481891303923 -0.0013634218224953438]  CenterOfMassUnits=mm  MomentsOfInertia=[0.00016543197172893975 0.0014334630955093895 0.0014333390308476422]  MomentsOfInertiaUnits=kg*mm^2  ProductsOfInertia=[-5.4062904633677868e-09 -1.3111174919527308e-07 6.0713893531177014e-07]  ProductsOfInertiaUnits=kg*mm^2  GraphicType=FromGeometry  MarkerShape=Sphere  MarkerSize=10  GraphicVisPropType=SimpleVisualProperties  GraphicDiffuseColor=[0.75294117647058822 0.75294117647058822 0.75294117647058822]  GraphicOpacity=1  GraphicSpecularColor=[0.5 0.5 0.5 1.0]  GraphicAmbientColor=[0.15 0.15 0.15 1.0]  GraphicEmissiveColor=[0.0 0.0 0.0 1.0]  GraphicShininess=75  DoExposeReferenceFrame=on  SerializedFrames=<Frames/>
  F : PMIOPort  Side=Left
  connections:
  Solid/RConn1 -- ReferenceFrame/RConn1 -- F/RConn1

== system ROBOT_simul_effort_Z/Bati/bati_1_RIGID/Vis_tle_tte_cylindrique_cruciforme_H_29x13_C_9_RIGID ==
  ReferenceFrame : sm_lib/Frames and Transforms/Reference Frame
  Solid : sm_lib/Body Elements/File Solid  ExtGeomFileName=/MATLAB Drive/Fichiers_Matlab_sujetA/Fichiers Matlab/STL/Vis a tole tete cylindrique cruciforme H 2-9x13 - C_Realiste_sldprt.STL  UnitType=Custom  ExtGeomFileUnits=mm  StepReaderType=HEX  ExportConvexHullGeometry=off  InertiaType=Custom  BasedOnType=Density  Density=1000  DensityUnits=kg/(m^3)  Mass=8.3821869835456372e-05  MassUnits=kg  CenterOfMass=[4.9478681581074904 0.00064910481891303923 -0.0013634218224953438]  CenterOfMassUnits=mm  MomentsOfInertia=[0.00016543197172893975 0.0014334630955093895 0.0014333390308476422]  MomentsOfInertiaUnits=kg*mm^2  ProductsOfInertia=[-5.4062904633677868e-09 -1.3111174919527308e-07 6.0713893531177014e-07]  ProductsOfInertiaUnits=kg*mm^2  GraphicType=FromGeometry  MarkerShape=Sphere  MarkerSize=10  GraphicVisPropType=SimpleVisualProperties  GraphicDiffuseColor=[0.75294117647058822 0.75294117647058822 0.75294117647058822]  GraphicOpacity=1  GraphicSpecularColor=[0.5 0.5 0.5 1.0]  GraphicAmbientColor=[0.15 0.15 0.15 1.0]  GraphicEmissiveColor=[0.0 0.0 0.0 1.0]  GraphicShininess=75  DoExposeReferenceFrame=on  SerializedFrames=<Frames/>
  F : PMIOPort  Side=Left
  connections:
  Solid/RConn1 -- ReferenceFrame/RConn1 -- F/RConn1

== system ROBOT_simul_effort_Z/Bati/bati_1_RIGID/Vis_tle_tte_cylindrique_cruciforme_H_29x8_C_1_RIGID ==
  ReferenceFrame : sm_lib/Frames and Transforms/Reference Frame
  Solid : sm_lib/Body Elements/File Solid  ExtGeomFileName=/MATLAB Drive/Fichiers_Matlab_sujetA/Fichiers Matlab/STL/Vis a tole tete cylindrique cruciforme H 2-9x8 - C_Realiste_sldprt.STL  UnitType=Custom  ExtGeomFileUnits=mm  StepReaderType=HEX  ExportConvexHullGeometry=off  InertiaType=Custom  BasedOnType=Density  Density=1000  DensityUnits=kg/(m^3)  Mass=6.1032951855347168e-05  MassUnits=kg  CenterOfMass=[2.8733410905856731 0.00094398948887705679 -0.0019024155537156445]  CenterOfMassUnits=mm  MomentsOfInertia=[0.0001480040782382925 0.00040137501597657324 0.00040131942245693811]  MomentsOfInertiaUnits=kg*mm^2  ProductsOfInertia=[3.5650623197794874e-09 -1.4668534891118034e-08 2.7820926592949074e-07]  ProductsOfInertiaUnits=kg*mm^2  GraphicType=FromGeometry  MarkerShape=Sphere  MarkerSize=10  GraphicVisPropType=SimpleVisualProperties  GraphicDiffuseColor=[0.75294117647058822 0.75294117647058822 0.75294117647058822]  GraphicOpacity=1  GraphicSpecularColor=[0.5 0.5 0.5 1.0]  GraphicAmbientColor=[0.15 0.15 0.15 1.0]  GraphicEmissiveColor=[0.0 0.0 0.0 1.0]  GraphicShininess=75  DoExposeReferenceFrame=on  SerializedFrames=<Frames/>
  F : PMIOPort  Side=Left
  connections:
  Solid/RConn1 -- ReferenceFrame/RConn1 -- F/RConn1

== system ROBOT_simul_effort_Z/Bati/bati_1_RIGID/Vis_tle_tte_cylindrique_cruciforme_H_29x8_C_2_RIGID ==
  ReferenceFrame : sm_lib/Frames and Transforms/Reference Frame
  Solid : sm_lib/Body Elements/File Solid  ExtGeomFileName=/MATLAB Drive/Fichiers_Matlab_sujetA/Fichiers Matlab/STL/Vis a tole tete cylindrique cruciforme H 2-9x8 - C_Realiste_sldprt.STL  UnitType=Custom  ExtGeomFileUnits=mm  StepReaderType=HEX  ExportConvexHullGeometry=off  InertiaType=Custom  BasedOnType=Density  Density=1000  DensityUnits=kg/(m^3)  Mass=6.1032951855347168e-05  MassUnits=kg  CenterOfMass=[2.8733410905856731 0.00094398948887705679 -0.0019024155537156445]  CenterOfMassUnits=mm  MomentsOfInertia=[0.0001480040782382925 0.00040137501597657324 0.00040131942245693811]  MomentsOfInertiaUnits=kg*mm^2  ProductsOfInertia=[3.5650623197794874e-09 -1.4668534891118034e-08 2.7820926592949074e-07]  ProductsOfInertiaUnits=kg*mm^2  GraphicType=FromGeometry  MarkerShape=Sphere  MarkerSize=10  GraphicVisPropType=SimpleVisualProperties  GraphicDiffuseColor=[0.75294117647058822 0.75294117647058822 0.75294117647058822]  GraphicOpacity=1  GraphicSpecularColor=[0.5 0.5 0.5 1.0]  GraphicAmbientColor=[0.15 0.15 0.15 1.0]  GraphicEmissiveColor=[0.0 0.0 0.0 1.0]  GraphicShininess=75  DoExposeReferenceFrame=on  SerializedFrames=<Frames/>
  F : PMIOPort  Side=Left
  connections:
  Solid/RConn1 -- ReferenceFrame/RConn1 -- F/RConn1

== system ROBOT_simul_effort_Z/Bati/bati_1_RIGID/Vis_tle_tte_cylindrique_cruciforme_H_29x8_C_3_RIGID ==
  ReferenceFrame : sm_lib/Frames and Transforms/Reference Frame
  Solid : sm_lib/Body Elements/File Solid  ExtGeomFileName=/MATLAB Drive/Fichiers_Matlab_sujetA/Fichiers Matlab/STL/Vis a tole tete cylindrique cruciforme H 2-9x8 - C_Realiste_sldprt.STL  UnitType=Custom  ExtGeomFileUnits=mm  StepReaderType=HEX  ExportConvexHullGeometry=off  InertiaType=Custom  BasedOnType=Density  Density=1000  DensityUnits=kg/(m^3)  Mass=6.1032951855347168e-05  MassUnits=kg  CenterOfMass=[2.8733410905856731 0.00094398948887705679 -0.0019024155537156445]  CenterOfMassUnits=mm  MomentsOfInertia=[0.0001480040782382925 0.00040137501597657324 0.00040131942245693811]  MomentsOfInertiaUnits=kg*mm^2  ProductsOfInertia=[3.5650623197794874e-09 -1.4668534891118034e-08 2.7820926592949074e-07]  ProductsOfInertiaUnits=kg*mm^2  GraphicType=FromGeometry  MarkerShape=Sphere  MarkerSize=10  GraphicVisPropType=SimpleVisualProperties  GraphicDiffuseColor=[0.75294117647058822 0.75294117647058822 0.75294117647058822]  GraphicOpacity=1  GraphicSpecularColor=[0.5 0.5 0.5 1.0]  GraphicAmbientColor=[0.15 0.15 0.15 1.0]  GraphicEmissiveColor=[0.0 0.0 0.0 1.0]  GraphicShininess=75  DoExposeReferenceFrame=on  SerializedFrames=<Frames/>
  F : PMIOPort  Side=Left
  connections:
  Solid/RConn1 -- ReferenceFrame/RConn1 -- F/RConn1
